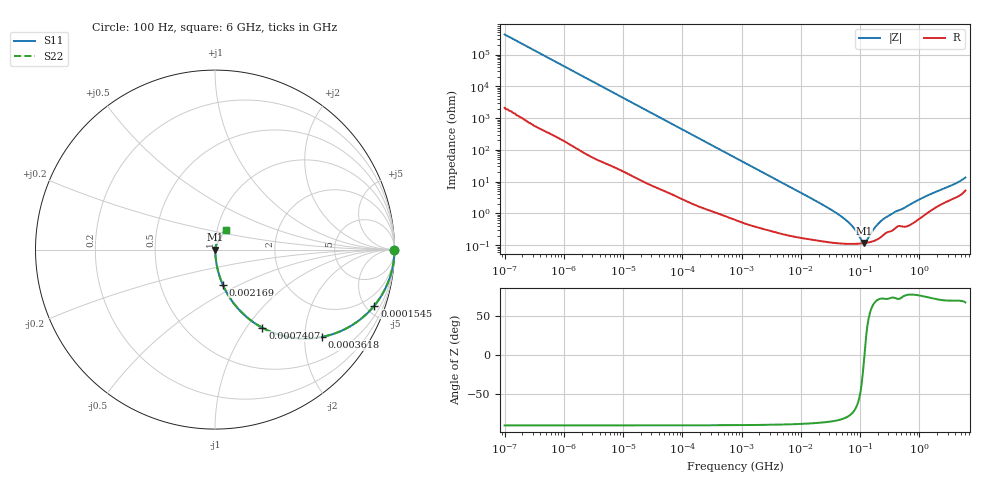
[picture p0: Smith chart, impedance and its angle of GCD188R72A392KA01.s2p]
!Murata Part Number: GCD188R72A392KA01
!These Parameters are Measured in Series Mode Connection
!Data Generated on Mar 13, 2026
!  o--ll--o
!Port1  Port2
!  o------o
!Operation Temp=25[degC], DC Bias Voltage=0[V]
!Freq. Start=100[Hz] Stop=6[GHz] 401[Steps]
# Hz S RI R 50
!Freq.(Hz) S11(Real) S11(Imag) S21(Real) S21(Imag) S12(Real) S12(Imag) S22(Real) S22(Imag)
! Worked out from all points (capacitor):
!   401 points, 100 Hz to 6 GHz, reference 50 ohm
!   read as one part in series: C = 3.71 nF near 109 Hz
!   lowest |Z| = 116 mohm at 116.7 MHz (marker M1)
!   series resonance near 118.6 MHz, so ESL is about 490 pH
!   S11 on the Smith chart (normalised r, x): 100 Hz: open; 154.5 kHz: 1.04, -5.67; 361.8 kHz: 1.02, -2.43; 740.7 kHz: 1.01, -1.19; 2.169 MHz: 1.01, -0.41; 6 GHz: 1.11, +0.25
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100  1 -0.000233  1.2e-06 0.000233  1.2e-06 0.000233  1 -0.000233
2008  1 -0.00464  4.05e-05 0.00464  4.05e-05 0.00464  1 -0.00464
40335  0.991 -0.0916  0.00898 0.0916  0.00898 0.0916  0.991 -0.0916
154540  0.8878 -0.3123  0.1122 0.3123  0.1122 0.3123  0.8878 -0.3123
231233  0.781 -0.4098  0.219 0.4098  0.219 0.4098  0.781 -0.4098
361830  0.5955 -0.4864  0.4045 0.4864  0.4045 0.4864  0.5955 -0.4864
740679  0.2644 -0.4357  0.7356 0.4357  0.7356 0.4357  0.2644 -0.4357
774597  0.2477 -0.4263  0.7523 0.4263  0.7523 0.4263  0.2477 -0.4263
1267578  0.1119 -0.3088  0.8881 0.3088  0.8881 0.3088  0.1119 -0.3088
2169299  0.0432 -0.1953  0.9568 0.1953  0.9568 0.1953  0.0432 -0.1953
5079039  0.00981 -0.0869  0.9902 0.0869  0.9902 0.0869  0.00981 -0.0869
1.555665e7  0.00229 -0.0285  0.9977 0.0285  0.9977 0.0285  0.00229 -0.0285
3.482834e7  0.00133 -0.012  0.9987 0.012  0.9987 0.012  0.00133 -0.012
5.699437e7  0.00114 -0.0062  0.9989 0.0062  0.9989 0.0062  0.00114 -0.0062
7.797396e7  0.00111 -0.00335  0.9989 0.00335  0.9989 0.00335  0.00111 -0.00335
1.066761e8  0.00113 -0.000827  0.9989 0.000827  0.9989 0.000827  0.00113 -0.000827
1.166697e8  0.00115 -0.000127  0.9988 0.000127  0.9988 0.000127  0.00115 -0.000127
1.275994e8  0.00118 0.000574  0.9988 -0.000574  0.9988 -0.000574  0.00118 0.000574
1.996653e8  0.00156 0.00431  0.9984 -0.00431  0.9984 -0.00431  0.00156 0.00431
3.124326e8  0.00272 0.00819  0.9973 -0.00819  0.9973 -0.00819  0.00272 0.00819
1.144649e9  0.00892 0.0295  0.9911 -0.0295  0.9911 -0.0295  0.00892 0.0295
6e9  0.063 0.1102  0.937 -0.1102  0.937 -0.1102  0.063 0.1102
